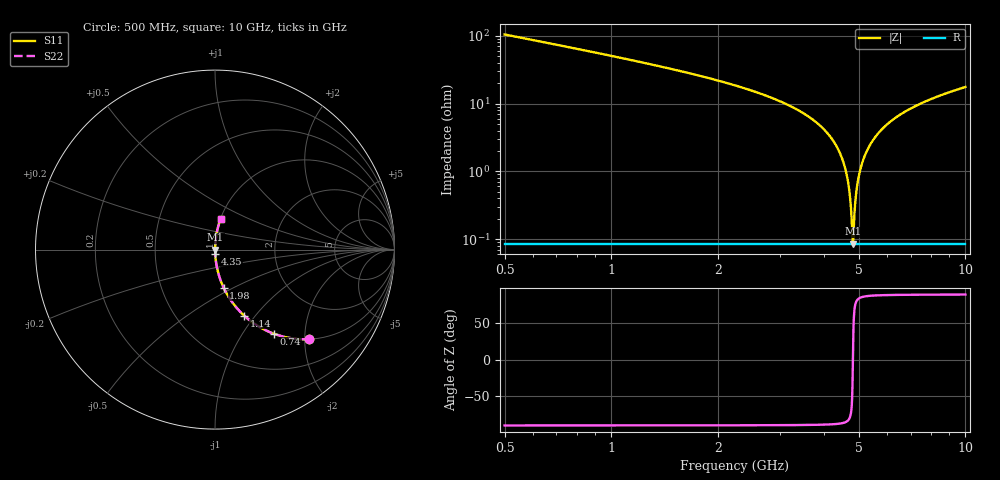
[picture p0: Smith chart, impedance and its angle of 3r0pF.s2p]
! Created Fri Jan 10 15:55:20 2014
# hz S db R 50
! 2 Port Network Data from SP1.SP block
! freq  dbS11  angS11  dbS21  angS21  dbS12  angS12  dbS22  angS22
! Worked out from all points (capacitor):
!   951 points, 500 MHz to 10 GHz, reference 50 ohm
!   read as one part in series: C = 3 pF near 540 MHz
!   lowest |Z| = 85.6 mohm at 4.81 GHz (marker M1)
!   series resonance near 4.812 GHz, so ESL is about 360 pH
!   S11 on the Smith chart (normalised r, x): 500 MHz: 1.00, -2.10; 740 MHz: 1.00, -1.40; 1.14 GHz: 1.00, -0.88; 1.98 GHz: 1.00, -0.45; 4.35 GHz: 1.00, -0.04; 10 GHz: 1.00, +0.35
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5e8  -2.81 -43.6  -3.23 46.4  -3.23 46.4  -2.81 -43.6
7.4e8  -4.84 -55.0  -1.74 35.0  -1.74 35.0  -4.84 -55.0
1.14e9  -7.92 -66.2  -0.77 23.7  -0.77 23.7  -7.92 -66.2
1.98e9  -13.27 -77.2  -0.22 12.5  -0.22 12.5  -13.27 -77.2
2.09e9  -13.91 -78.1  -0.19 11.6  -0.19 11.6  -13.91 -78.1
3.67e9  -24.39 -85.7  -0.02 3.5  -0.02 3.5  -24.39 -85.7
4.06e9  -28.49 -86.6  -0.01 2.2  -0.01 2.2  -28.49 -86.6
4.35e9  -33.03 -86.5  -0.01 1.3  -0.01 1.3  -33.03 -86.5
4.52e9  -37.18 -85.7  -0.01 0.8  -0.01 0.8  -37.18 -85.7
4.64e9  -41.85 -83.5  -0.01 0.5  -0.01 0.5  -41.85 -83.5
4.71e9  -46.36 -79.6  -0.01 0.3  -0.01 0.3  -46.36 -79.6
4.78e9  -55.35 -60.1  -0.01 0.1  -0.01 0.1  -55.35 -60.1
4.81e9  -61.35 -7.0  -0.01 0.0  -0.01 0.0  -61.35 -7.0
4.84e9  -56.34 56.1  -0.01 -0.1  -0.01 -0.1  -56.34 56.1
4.91e9  -46.92 78.9  -0.01 -0.3  -0.01 -0.3  -46.92 78.9
4.98e9  -42.39 83.1  -0.01 -0.4  -0.01 -0.4  -42.39 83.1
5.09e9  -38.14 85.4  -0.01 -0.7  -0.01 -0.7  -38.14 85.4
5.25e9  -34.33 86.4  -0.01 -1.1  -0.01 -1.1  -34.33 86.4
5.85e9  -27.28 86.4  -0.02 -2.5  -0.02 -2.5  -27.28 86.4
6.84e9  -22.07 84.9  -0.03 -4.5  -0.03 -4.5  -22.07 84.9
8.42e9  -17.81 82.2  -0.08 -7.4  -0.08 -7.4  -17.81 82.2
1e10  -15.23 79.7  -0.14 -10.0  -0.14 -10.0  -15.23 79.7
